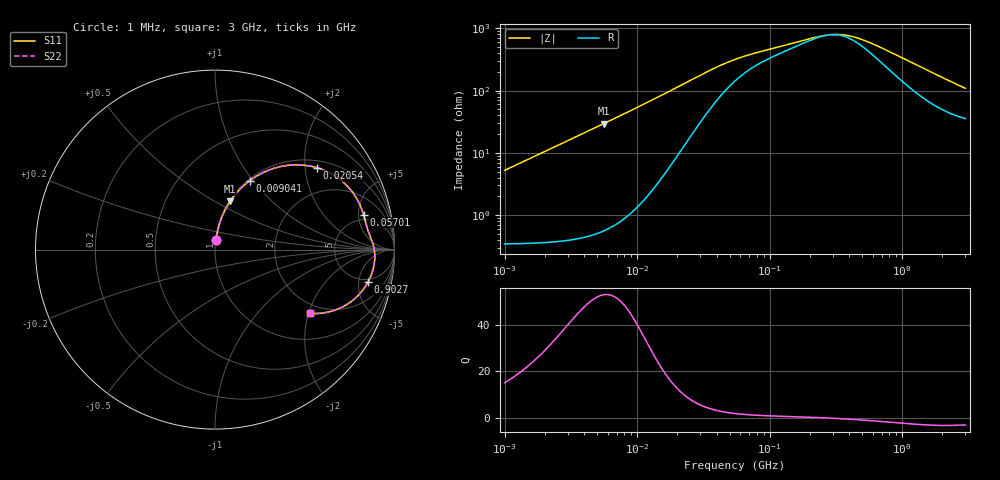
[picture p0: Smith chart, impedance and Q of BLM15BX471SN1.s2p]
! BLM15BX471SN1
# Hz S RI R 50
!Freq.(Hz) S11(Real) S11(Imag) S21(Real) S21(Imag) S12(Real) S12(Imag) S22(Real) S22(Imag)
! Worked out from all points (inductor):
!   401 points, 1 MHz to 3 GHz, reference 50 ohm
!   read as one part in series: L = 833 nH near 1.041 MHz
!   highest Q = 52.8 at 5.592 MHz (marker M1), where L = 839 nH
!   self-resonance near 286.9 MHz
!   S11 on the Smith chart (normalised r, x): 1 MHz: 1.01, +0.10; 9.041 MHz: 1.02, +0.97; 20.54 MHz: 1.19, +2.32; 57.01 MHz: 4.09, +5.75; 902.7 MHz: 4.42, -6.65; 3 GHz: 1.71, -2.06
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1000000  0.00615 0.0518  0.9939 -0.0518  0.9939 -0.0518  0.00615 0.0518
2055611  0.015 0.1056  0.985 -0.1056  0.985 -0.1056  0.015 0.1056
3823119  0.0425 0.1914  0.9575 -0.1914  0.9575 -0.1914  0.0425 0.1914
5592179  0.0843 0.2685  0.9157 -0.2685  0.9157 -0.2685  0.0843 0.2685
9040831  0.1944 0.3846  0.8056 -0.3846  0.8056 -0.3846  0.1944 0.3846
1.461624e7  0.3959 0.468  0.6041 -0.468  0.6041 -0.468  0.3959 0.468
2.054061e7  0.57 0.4555  0.43 -0.4555  0.43 -0.4555  0.57 0.4555
2.611722e7  0.6768 0.4052  0.3232 -0.4052  0.3232 -0.4052  0.6768 0.4052
3.254976e7  0.7482 0.3421  0.2518 -0.3421  0.2518 -0.3421  0.7482 0.3421
4.138676e7  0.7963 0.272  0.2037 -0.272  0.2037 -0.272  0.7963 0.272
5.477226e7  0.8249 0.2034  0.1751 -0.2034  0.1751 -0.2034  0.8249 0.2034
5.700937e7  0.8275 0.1952  0.1725 -0.1952  0.1725 -0.1952  0.8275 0.1952
8.854986e7  0.8465 0.1254  0.1535 -0.1254  0.1535 -0.1254  0.8465 0.1254
2.094008e8  0.879 0.0357  0.121 -0.0357  0.121 -0.0357  0.879 0.0357
2.884452e8  0.8876 -0.000652  0.1124 0.000652  0.1124 0.000652  0.8876 -0.000652
3.817355e8  0.8904 -0.0365  0.1096 0.0365  0.1096 0.0365  0.8904 -0.0365
5.154121e8  0.887 -0.0802  0.113 0.0802  0.113 0.0802  0.887 -0.0802
8.005644e8  0.8642 -0.157  0.1358 0.157  0.1358 0.157  0.8642 -0.157
9.0272e8  0.8526 -0.1808  0.1474 0.1808  0.1474 0.1808  0.8526 -0.1808
1.54974e9  0.7549 -0.2923  0.2451 0.2923  0.2451 0.2923  0.7549 -0.2923
2.177892e9  0.649 -0.3435  0.351 0.3435  0.351 0.3435  0.649 -0.3435
3e9  0.5315 -0.3555  0.4685 0.3555  0.4685 0.3555  0.5315 -0.3555
